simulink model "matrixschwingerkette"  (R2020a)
settings: Solver=ode45  StartTime=0.0  StopTime=10.0  RelTol=1e-3  EnableMultiTasking=on

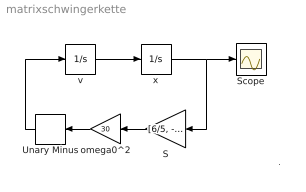
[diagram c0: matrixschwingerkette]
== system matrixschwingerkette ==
  note: .
  S : Gain  Gain=[6/5, -1/5; -1/5, 6/5]  Multiplication=Matrix(K*u)  SaturateOnIntegerOverflow=on
  Scope : Scope
  Unary Minus : UnaryMinus
  omega0^2 : Gain  Gain=30  SaturateOnIntegerOverflow=on
  v : Integrator  InitialCondition=[0 0]
  x : Integrator  InitialCondition=[1 0]
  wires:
  v/1 -> x/1
  x/1 -> S/1, Scope/1
  S/1 -> omega0^2/1
  omega0^2/1 -> Unary Minus/1
  Unary Minus/1 -> v/1
